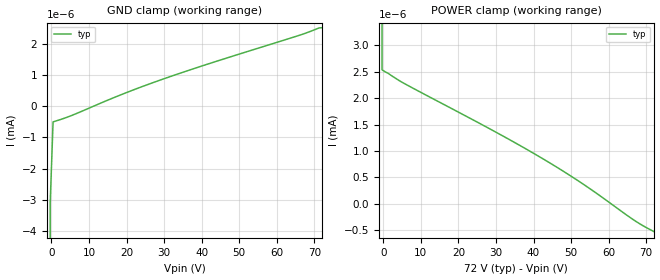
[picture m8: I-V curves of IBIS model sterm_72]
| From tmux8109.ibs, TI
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| sterm_72
[Model]   sterm_72
Model_type   Terminator
|   typ   min   max
C_comp   4.014581e-12   NA   NA
[Voltage Range]   72   NA   NA
[Temperature Range]   27   NA   NA
[Power Clamp Reference]   72   NA   NA
[GND Clamp Reference]   0   NA   NA
[GND Clamp]
|   Voltage   I(typ)   I(min)   I(max)
-5V       -1.133A    NA         NA
-1.111V   -35.61mA   NA         NA
-333.3mV  -3.131nA   NA         NA
444.4mV   -505.4pA   NA         NA
5.111V    -313.9pA   NA         NA
18.33V    352.5pA    NA         NA
30V       874.8pA    NA         NA
66.56V    2.284nA    NA         NA
71.22V    2.497nA    NA         NA
72V       2.506nA    NA         NA
[POWER Clamp]
|   Voltage   I(typ)   I(min)   I(max)
-5V       744mA      NA         NA
-1.111V   26.13mA    NA         NA
-333.3mV  2.538nA    NA         NA
5.111V    2.297nA    NA         NA
29.22V    1.387nA    NA         NA
42.44V    856pA      NA         NA
53.33V    368.5pA    NA         NA
67.33V    -334.5pA   NA         NA
72V       -522.1pA   NA         NA
